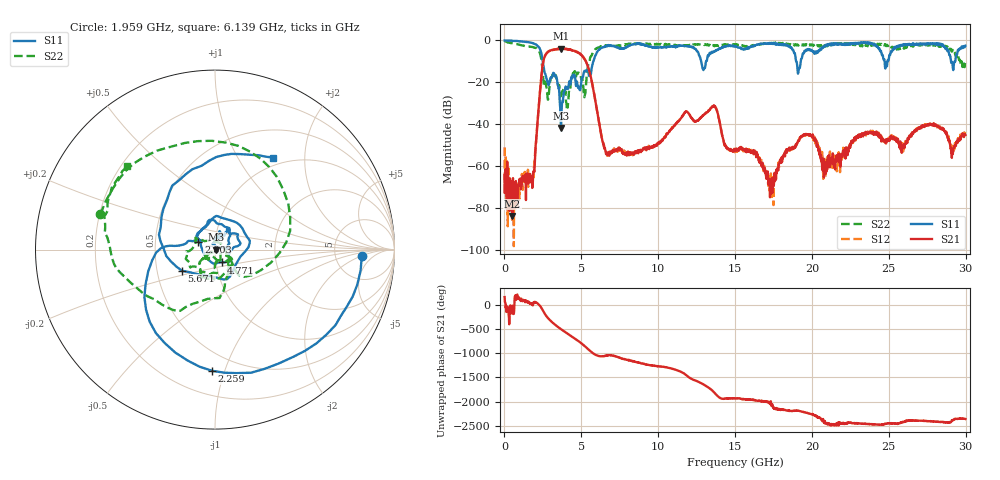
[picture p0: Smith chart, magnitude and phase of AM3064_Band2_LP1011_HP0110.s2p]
# Hz S DB R 50.0
!freq dBS11 angS11 dBS21 angS21 dBS12 angS12 dBS22 angS22
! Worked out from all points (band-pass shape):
!   1600 points, 10 MHz to 29.98 GHz, reference 50 ohm
!   highest |S21| = -3.91 dB at 3.703 GHz (marker M1); lowest = -83.8 dB at 516.1 MHz (marker M2)
!   |S21| within 3 dB of the highest: 2.669 GHz to 4.998 GHz (2.328 GHz wide, 60.7 % of centre)
!   lowest |S11| = -41.8 dB at 3.684 GHz (marker M3), VSWR 1.02, Z = 50.8 + j0.0459 ohm
!   |S11| at or under -10 dB: 2.493 GHz to 5.775 GHz (3.283 GHz wide, 79.4 % of centre); 12.8 GHz to 13.12 GHz (318.1 MHz wide, 2.45 % of centre); 18.98 GHz to 19.27 GHz (288.6 MHz wide, 1.51 % of centre)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
!   |S22| runs from -32.8 to -0.2 dB; largest |S21 - S12| = 0.013
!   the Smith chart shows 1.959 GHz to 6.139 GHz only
!   S11 on the Smith chart (normalised r, x): 1.959 GHz: 9.62, -2.04; 2.259 GHz: 0.37, -0.91; 2.803 GHz: 0.83, +0.07; 4.771 GHz: 1.06, -0.15; 5.671 GHz: 0.67, -0.17; 6.139 GHz: 0.88, +1.42
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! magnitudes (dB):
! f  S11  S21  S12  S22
! 10 MHz  0.0  -64.3  -51.1  -0.2
! 516.1 MHz  -0.2  -83.8  -68.3  -1.4
! 1.959 GHz  -1.7  -60.7  -57.7  -3.5
! 2.259 GHz  -3.4  -29.1  -29.0  -5.2
! 2.803 GHz  -19.8  -5.7  -5.6  -26.9
! 3.29 GHz  -16.7  -4.3  -4.2  -17.1
! 3.684 GHz  -41.8  -4.0  -3.9  -23.8
! 3.703 GHz  -34.7  -3.9  -4.0  -23.4
! 4.771 GHz  -21.9  -5.9  -5.7  -16.0
! 5.015 GHz  -18.4  -7.1  -7.1  -18.8
! 5.671 GHz  -13.2  -19.4  -19.3  -7.2
! 6.139 GHz  -4.4  -38.5  -38.5  -3.4
! 6.72 GHz  -2.5  -53.6  -54.5  -2.3
! 10 GHz  -3.4  -49.1  -49.4  -1.9
! 13.6 GHz  -5.3  -31.6  -31.2  -2.6
! 15 GHz  -2.7  -53.0  -53.3  -1.8
! 17.35 GHz  -1.3  -71.9  -69.2  -1.3
! 19.11 GHz  -15.5  -48.2  -48.0  -2.4
! 19.99 GHz  -4.7  -46.0  -45.7  -1.9
! 20.85 GHz  -2.8  -58.2  -58.6  -2.6
! 25 GHz  -9.1  -47.3  -47.5  -2.3
! 29.98 GHz  -2.5  -45.1  -44.6  -10.3
